(* Logix 5000 AddOnInstructionDefinition export GracoCore_DecodeDateTime; software revision 32.04; part 3 of 4 *)

ADD_ON_INSTRUCTION GracoPd2kDual_ReadFlushSeq   (* revision 1.0 *)
// Help:
// Returns the current configuration values for a flush sequence number.
// Values outside of acceptable ranges will result in an error being raised.
// State Codes:
// * 0000 (IDLE) - Idle
// * 1000 (BUSY) - Busy
// * 2000 (DONE) - Done
// * 4000 (ABORT) - Command overwritten by another process
// * 8000 (ERROR) - Flush sequence number out of range
// * 8001 (ERROR) - Timeout waiting for DCS registers
// * 8002 (ERROR) - Command unsuccessful
// * 8003 (ERROR) - Unhandled internal error
VAR_INPUT
   i_execute : BOOL; {visible}   // Execute command
   i_flushSeqNum : DINT; {visible}   // Flush sequence number
END_VAR
VAR_OUTPUT
   o_gunPurgeTime : DINT; {access Read Only, visible}   // Gun purge time (s)
   o_initialFlushVol : DINT; {access Read Only, visible}   // Initial flush volume (cc)
   o_finalFlushVol : DINT; {access Read Only, visible}   // Final flush volume (cc)
   o_numWashCycles : DINT; {access Read Only, visible}   // Number of wash cycles
   o_strokesPerWashCycle : DINT; {access Read Only, visible}   // Strokes per wash cycle
   o_busy : BOOL; {access Read Only, visible}   // Busy flag
   o_done : BOOL; {access Read Only, visible}   // Done flag
   o_aborted : BOOL; {access Read Only, visible}   // Aborted flag
   o_error : BOOL; {access Read Only, visible}   // Error flag
END_VAR
VAR_IN_OUT
   io_moduleStatus : DINT[62]; {required}   // Data from device to PLC
   io_moduleCmds : DINT[30]; {required}   // Data from PLC to device
END_VAR
VAR_OUTPUT
   o_state : DINT; {access Read Only, visible}   // Command state
END_VAR
VAR
   sendDCSInst : GracoPd2kDual_SendDCS; {access None}   // SendDCS instruction
END_VAR

ROUTINE Logic   (* ladder *)
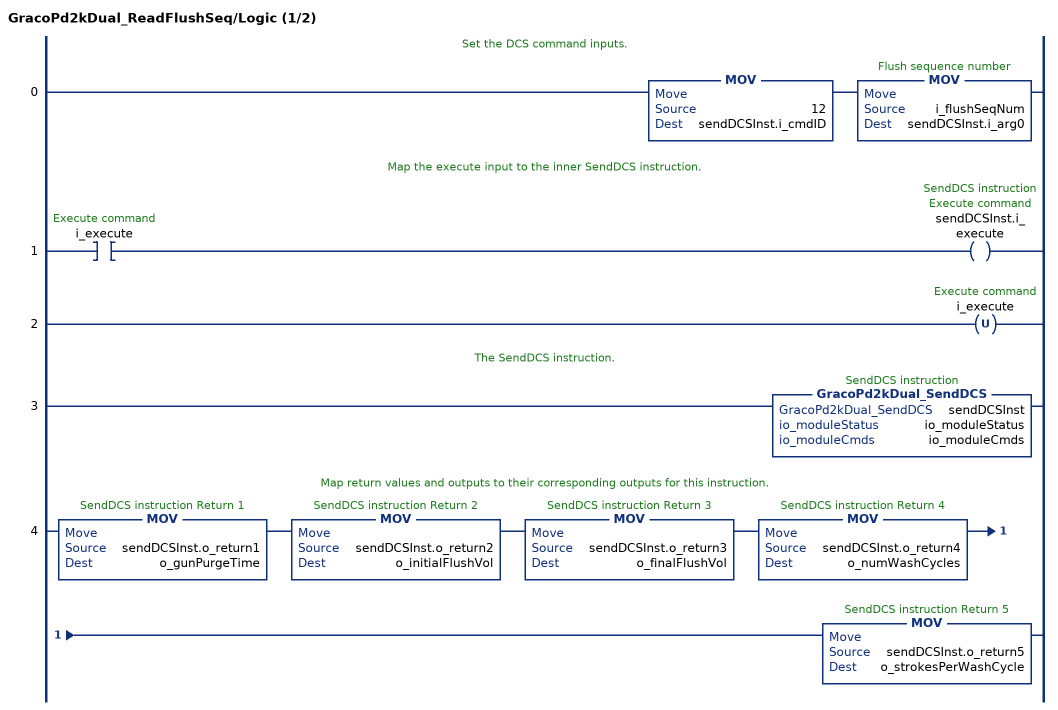
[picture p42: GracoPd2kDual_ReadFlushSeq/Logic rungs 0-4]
   // Set the DCS command inputs.
   0: MOV(12,sendDCSInst.i_cmdID)MOV(i_flushSeqNum,sendDCSInst.i_arg0);
   // Map the execute input to the inner SendDCS instruction.
   1: XIC(i_execute)OTE(sendDCSInst.i_execute);
   2: OTU(i_execute);
   // The SendDCS instruction.
   3: GracoPd2kDual_SendDCS(sendDCSInst,io_moduleStatus,io_moduleCmds);
   // Map return values and outputs to their corresponding outputs for this instruction.
   4: MOV(sendDCSInst.o_return1,o_gunPurgeTime)MOV(sendDCSInst.o_return2,o_initialFlushVol)MOV(sendDCSInst.o_return3,o_finalFlushVol)MOV(sendDCSInst.o_return4,o_numWashCycles)MOV(sendDCSInst.o_return5,o_strokesPerWashCycle);
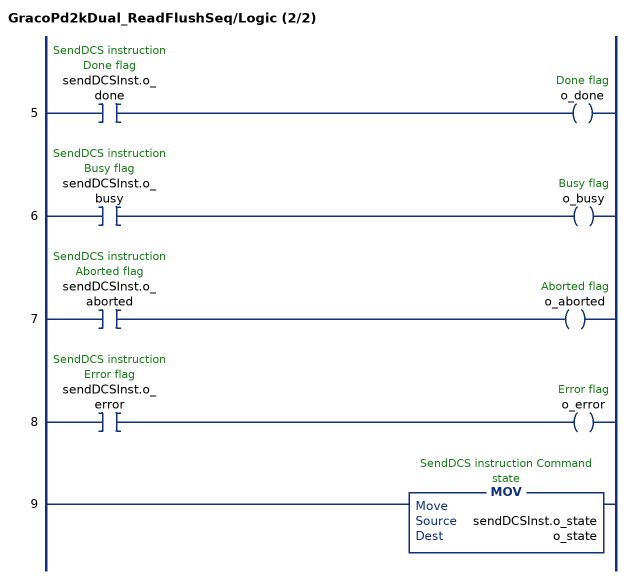
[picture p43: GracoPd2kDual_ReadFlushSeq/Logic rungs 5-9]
   5: XIC(sendDCSInst.o_done)OTE(o_done);
   6: XIC(sendDCSInst.o_busy)OTE(o_busy);
   7: XIC(sendDCSInst.o_aborted)OTE(o_aborted);
   8: XIC(sendDCSInst.o_error)OTE(o_error);
   9: MOV(sendDCSInst.o_state,o_state);
END_ROUTINE
END_ADD_ON_INSTRUCTION

ADD_ON_INSTRUCTION GracoPd2kDual_ReadGrandTotals   (* revision 1.0 *)
// Help:
// Returns the material usage statistics of the system.
// State Codes:
// * 0000 (IDLE) - Idle
// * 1000 (BUSY) - Busy
// * 2000 (DONE) - Done
// * 4000 (ABORT) - Command overwritten by another process
// * 8001 (ERROR) - Timeout waiting for DCS registers
// * 8002 (ERROR) - Command unsuccessful
// * 8003 (ERROR) - Unhandled internal error
VAR_INPUT
   i_execute : BOOL; {visible}   // Execute command
END_VAR
VAR_OUTPUT
   o_materialA : DINT; {access Read Only, visible}   // Material A total volume (gal)
   o_materialB : DINT; {access Read Only, visible}   // Material B total volume (gal)
   o_materialAB : DINT; {access Read Only, visible}   // Materials A+B total volume (gal)
   o_solvent : DINT; {access Read Only, visible}   // Solvent volume (gal)
   o_busy : BOOL; {access Read Only, visible}   // Busy flag
   o_done : BOOL; {access Read Only, visible}   // Done flag
   o_aborted : BOOL; {access Read Only, visible}   // Aborted flag
   o_error : BOOL; {access Read Only, visible}   // Error flag
   o_state : DINT; {access Read Only, visible}   // Command state
END_VAR
VAR_IN_OUT
   io_moduleStatus : DINT[62]; {required}   // Data from device to PLC
   io_moduleCmds : DINT[30]; {required}   // Data from PLC to device
END_VAR
VAR
   sendDCSInst : GracoPd2kDual_SendDCS; {access None}   // SendDCS instruction
END_VAR

ROUTINE Logic   (* ladder *)
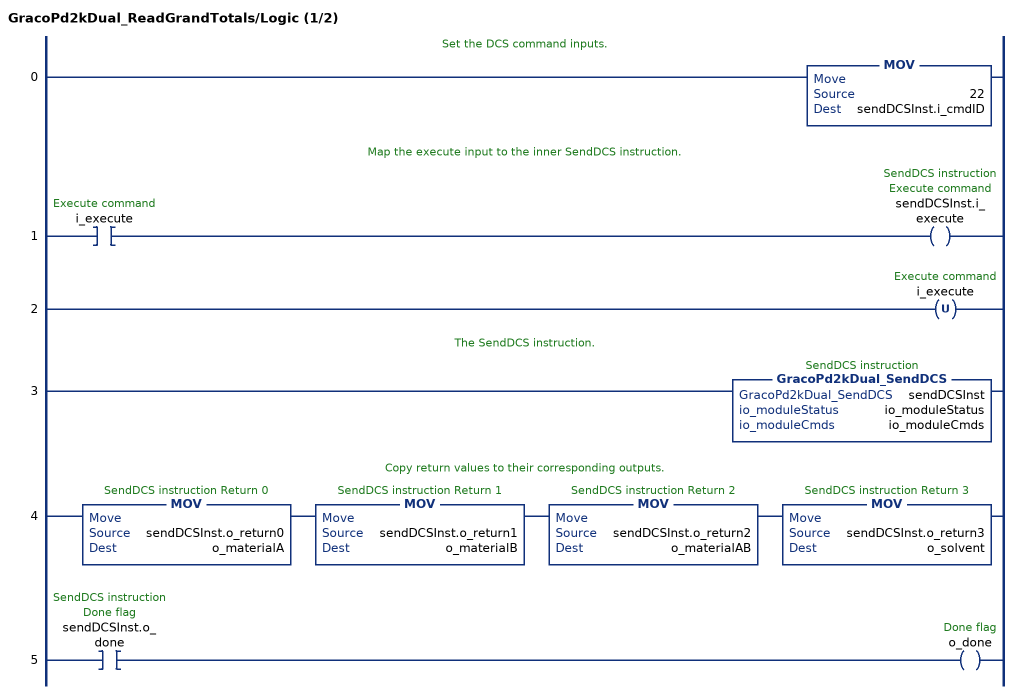
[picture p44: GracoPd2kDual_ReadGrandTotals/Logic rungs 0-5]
   // Set the DCS command inputs.
   0: MOV(22,sendDCSInst.i_cmdID);
   // Map the execute input to the inner SendDCS instruction.
   1: XIC(i_execute)OTE(sendDCSInst.i_execute);
   2: OTU(i_execute);
   // The SendDCS instruction.
   3: GracoPd2kDual_SendDCS(sendDCSInst,io_moduleStatus,io_moduleCmds);
   // Copy return values to their corresponding outputs.
   4: MOV(sendDCSInst.o_return0,o_materialA)MOV(sendDCSInst.o_return1,o_materialB)MOV(sendDCSInst.o_return2,o_materialAB)MOV(sendDCSInst.o_return3,o_solvent);
   5: XIC(sendDCSInst.o_done)OTE(o_done);
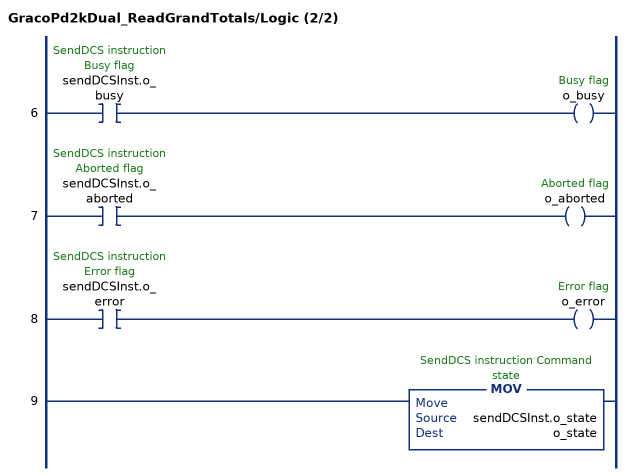
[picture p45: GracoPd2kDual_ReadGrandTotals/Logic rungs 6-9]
   6: XIC(sendDCSInst.o_busy)OTE(o_busy);
   7: XIC(sendDCSInst.o_aborted)OTE(o_aborted);
   8: XIC(sendDCSInst.o_error)OTE(o_error);
   9: MOV(sendDCSInst.o_state,o_state);
END_ROUTINE
END_ADD_ON_INSTRUCTION

ADD_ON_INSTRUCTION GracoPd2kDual_ReadRecipe   (* revision 1.0 *)
// Help:
// Returns the current configuration values for a recipe number.
// If mixUnitNum or recipeNum is out of range, an error will be raised.
// State Codes:
// * 0000 (IDLE) - Idle
// * 1000 (BUSY) - Busy
// * 2000 (DONE) - Done
// * 4000 (ABORT) - Command overwritten by another process
// * 8000 (ERROR) - Invalid input ranges
// * 8001 (ERROR) - Timeout waiting for DCS registers
// * 8002 (ERROR) - Command unsuccessful
// * 8003 (ERROR) - Unhandled internal error
VAR_INPUT
   i_execute : BOOL; {visible}   // Execute command
   i_mixUnitNum : DINT; {visible}   // Mix unit number (1-2)
   i_recipeNum : DINT; {visible}   // Recipe number (0-30)
END_VAR
VAR_OUTPUT
   o_materialA : DINT; {access Read Only, visible}   // Material A
   o_materialB : DINT; {access Read Only, visible}   // Material B
   o_flushSeqA : DINT; {access Read Only, visible}   // Flush sequence A
   o_flushSeqB : DINT; {access Read Only, visible}   // Flush sequence B
   o_mixRatioSP : REAL; {access Read Only, visible}   // Mix ratio setpoint (A:B)
   o_potLifeTimeSP : DINT; {access Read Only, visible}   // Pot life time setpoint (min)
   o_mixPressureTol : DINT; {access Read Only, visible}   // Mix pressure tolerance (%)
   o_busy : BOOL; {access Read Only, visible}   // Busy flag
   o_done : BOOL; {access Read Only, visible}   // Done flag
   o_aborted : BOOL; {access Read Only, visible}   // Aborted flag
   o_error : BOOL; {access Read Only, visible}   // Error flag
   o_state : DINT; {access Read Only, visible}   // Command state
END_VAR
VAR_IN_OUT
   io_moduleStatus : DINT[62]; {required}   // Data from device to PLC
   io_moduleCmds : DINT[30]; {required}   // Data from PLC to device
END_VAR
VAR
   sendDCSInst : GracoPd2kDual_SendDCS; {access None}   // SendDCS instruction
END_VAR

ROUTINE Logic   (* ladder *)
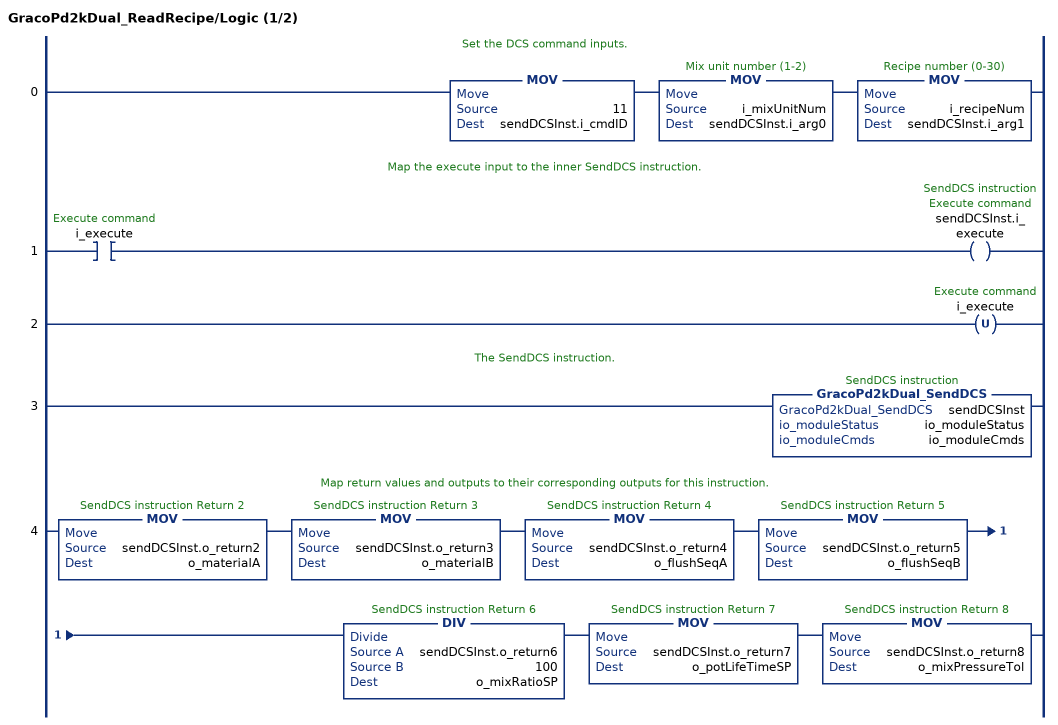
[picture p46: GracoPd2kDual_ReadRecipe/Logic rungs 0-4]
   // Set the DCS command inputs.
   0: MOV(11,sendDCSInst.i_cmdID)MOV(i_mixUnitNum,sendDCSInst.i_arg0)MOV(i_recipeNum,sendDCSInst.i_arg1);
   // Map the execute input to the inner SendDCS instruction.
   1: XIC(i_execute)OTE(sendDCSInst.i_execute);
   2: OTU(i_execute);
   // The SendDCS instruction.
   3: GracoPd2kDual_SendDCS(sendDCSInst,io_moduleStatus,io_moduleCmds);
   // Map return values and outputs to their corresponding outputs for this instruction.
   4: MOV(sendDCSInst.o_return2,o_materialA)MOV(sendDCSInst.o_return3,o_materialB)MOV(sendDCSInst.o_return4,o_flushSeqA)MOV(sendDCSInst.o_return5,o_flushSeqB)DIV(sendDCSInst.o_return6,100,o_mixRatioSP)MOV(sendDCSInst.o_return7,o_potLifeTimeSP)MOV(sendDCSInst.o_return8,o_mixPressureTol);
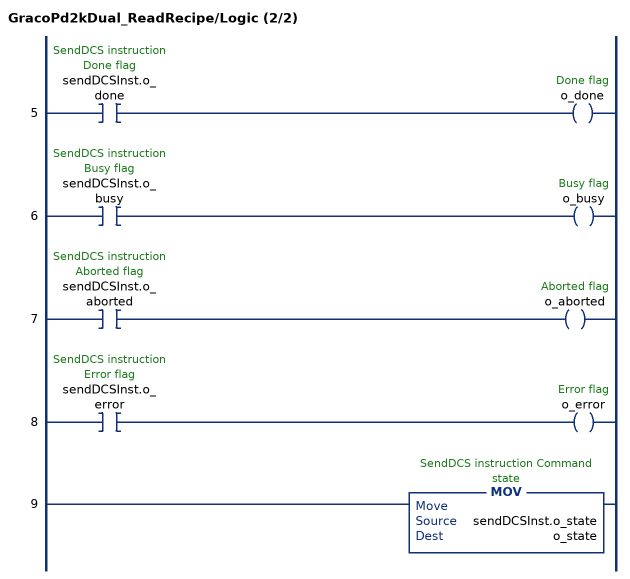
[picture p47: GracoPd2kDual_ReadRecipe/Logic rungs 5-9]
   5: XIC(sendDCSInst.o_done)OTE(o_done);
   6: XIC(sendDCSInst.o_busy)OTE(o_busy);
   7: XIC(sendDCSInst.o_aborted)OTE(o_aborted);
   8: XIC(sendDCSInst.o_error)OTE(o_error);
   9: MOV(sendDCSInst.o_state,o_state);
END_ROUTINE
END_ADD_ON_INSTRUCTION

ADD_ON_INSTRUCTION GracoPd2kDual_RecipeChange   (* revision 1.0 *)
// Help:
// Performs a recipe change operation.
// This command monitors the system throughout the operation, returning state codes depending on various conditions.
// State Codes:
// * 0000 (IDLE) - Idle
// * 1000 (BUSY) - busy
// * 2000 (DONE) - Complete
// * 4000 (ABORT) - Command overwritten by another process
// * 8000 (ERROR) - Invalid input ranges
// * 8001 (ERROR) - Could not start, pumps are turned off
// * 8002 (ERROR) - Another recipe change is currently in progress
// * 8003 (ERROR) - Could not start, a system alarm in active
// * 8004 (ERROR) - Could not start, another operation is in progress
// * 8006 (ERROR) - Timeout waiting for DCS registers
// * 8007 (ERROR) - Alarm occurred
// * 8008 (ERROR) - Unexpected system mode
// * 8009 (ERROR) - Timeout occurred waiting for fill to start
// * 800A (ERROR) - Timeout occurred waiting for mixing to start
// * 800B (ERROR) - Timeout occurred waiting for system command register
VAR_INPUT
   i_execute : BOOL; {visible}   // Execute command
   i_recipeNum : DINT; {visible}   // Recipe number
   i_mixUnitNum : DINT; {visible}   // Mix unit number
END_VAR
VAR_IN_OUT
   io_moduleStatus : DINT[62]; {required}   // Data from device to PLC
   io_moduleCmds : DINT[30]; {required}   // Data from PLC to device
END_VAR
VAR_OUTPUT
   o_busy : BOOL; {access Read Only, visible}   // Busy flag
   o_done : BOOL; {access Read Only, visible}   // Done flag
   o_aborted : BOOL; {access Read Only, visible}   // Aborted flag
   o_error : BOOL; {access Read Only, visible}   // Error flag
   o_state : DINT; {access Read Only, visible}   // Command state
END_VAR
VAR
   _systemMode : DINT; {access None}   // Current system mode
   rateLimitTmr : TIMER := (PRE := 250); {access None}   // Rate limit timer
   state_writeGotoRecipe : DINT; {access None}
   state_writeCmd : DINT; {access None}
   state_rateLimit : DINT; {access None}
   state_errorUnknownSystemMode : DINT; {access None}
   state_errorSystemInUse : DINT; {access None}
   state_errorRecipeChangeInProgress : DINT; {access None}
   state_errorPowerIsOff : DINT; {access None}
   state_errorIncomplete : DINT; {access None}
   state_errorAnotherOperation : DINT; {access None}
   state_errorAlarmOccurred : DINT; {access None}
   state_errorAlarmActive : DINT; {access None}
   state_done : DINT; {access None}
   state_checkSysState : DINT; {access None}
   state_await : DINT; {access None}
   state_aborted : DINT; {access None}
   recipeCmdConstant : DINT; {access None}
   _nextState : DINT; {access None}
   recipeChangeInProgress : BOOL; {access None}
   inStandby : BOOL; {access None}
   knownSystemMode : BOOL; {access None}
   systemPowerIsOff : BOOL; {access None}
   alarmIsActive : BOOL; {access None}
   systemInMixReadyMode : BOOL; {access None}
   systemInFillReadyMode : BOOL; {access None}
   systemInMixNotReadyMode : BOOL; {access None}
   state_checkInputs : DINT; {access None}
   _mixUnitNum : DINT; {access None}   // Mix unit number (internal)
   inUseTmr : TIMER := (PRE := 5000); {access None}
   recipeNumDelayTmr : TIMER := (PRE := 200); {access None}
   startedTmr : TIMER := (PRE := 2000); {access None}
   recipeChangeCompleted : BOOL; {access None}
   incompleteStuckInFillReady : BOOL; {access None}
   incompleteMixNotReady : BOOL; {access None}
   incompleteUnexpectedMode : BOOL; {access None}
   execute_ons : BOOL; {access None}
   mixUnitNumIsValid : BOOL; {access None}
   state_errorInvalidMixUnitNum : DINT; {access None}
   _currentSystemCmd : DINT; {access None}
   _currentNextRecipeCmd : DINT; {access None}
END_VAR

ROUTINE Logic   (* ladder *)
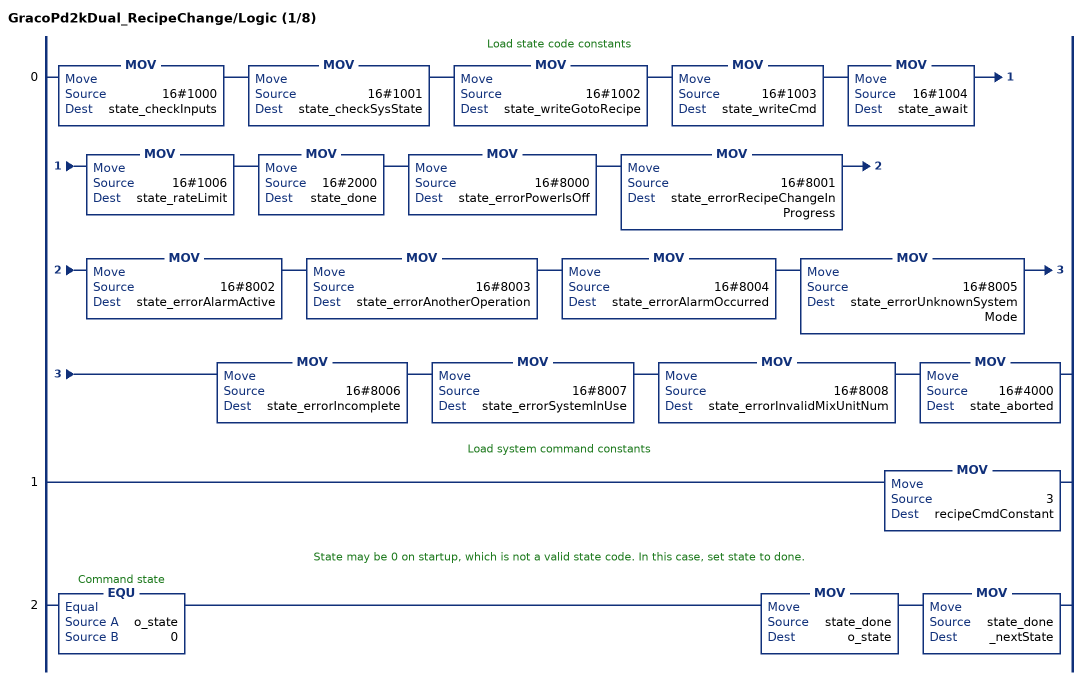
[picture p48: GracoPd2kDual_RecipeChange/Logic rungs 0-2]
   // Load state code constants
   0: MOV(16#1000,state_checkInputs)MOV(16#1001,state_checkSysState)MOV(16#1002,state_writeGotoRecipe)MOV(16#1003,state_writeCmd)MOV(16#1004,state_await)MOV(16#1006,state_rateLimit)MOV(16#2000,state_done)MOV(16#8000,state_errorPowerIsOff)MOV(16#8001,state_errorRecipeChangeInProgress)MOV(16#8002,state_errorAlarmActive)MOV(16#8003,state_errorAnotherOperation)MOV(16#8004,state_errorAlarmOccurred)MOV(16#8005,state_errorUnknownSystemMode)MOV(16#8006,state_errorIncomplete)MOV(16#8007,state_errorSystemInUse)MOV(16#8008,state_errorInvalidMixUnitNum)MOV(16#4000,state_aborted);
   // Load system command constants
   1: MOV(3,recipeCmdConstant);
   // State may be 0 on startup, which is not a valid state code. In this case, set state to done.
   2: EQU(o_state,0)MOV(state_done,o_state)MOV(state_done,_nextState);
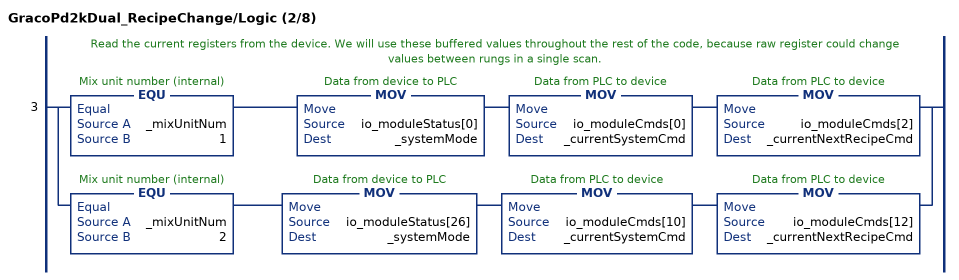
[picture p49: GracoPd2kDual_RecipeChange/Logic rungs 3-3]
   // Read the current registers from the device. We will use these buffered values throughout the rest of the code, because raw register could change values between rungs in a single scan.
   3: [EQU(_mixUnitNum,1) MOV(io_moduleStatus[0],_systemMode) MOV(io_moduleCmds[0],_currentSystemCmd) MOV(io_moduleCmds[2],_currentNextRecipeCmd) ,EQU(_mixUnitNum,2) MOV(io_moduleStatus[26],_systemMode) MOV(io_moduleCmds[10],_currentSystemCmd) MOV(io_moduleCmds[12],_currentNextRecipeCmd) ];
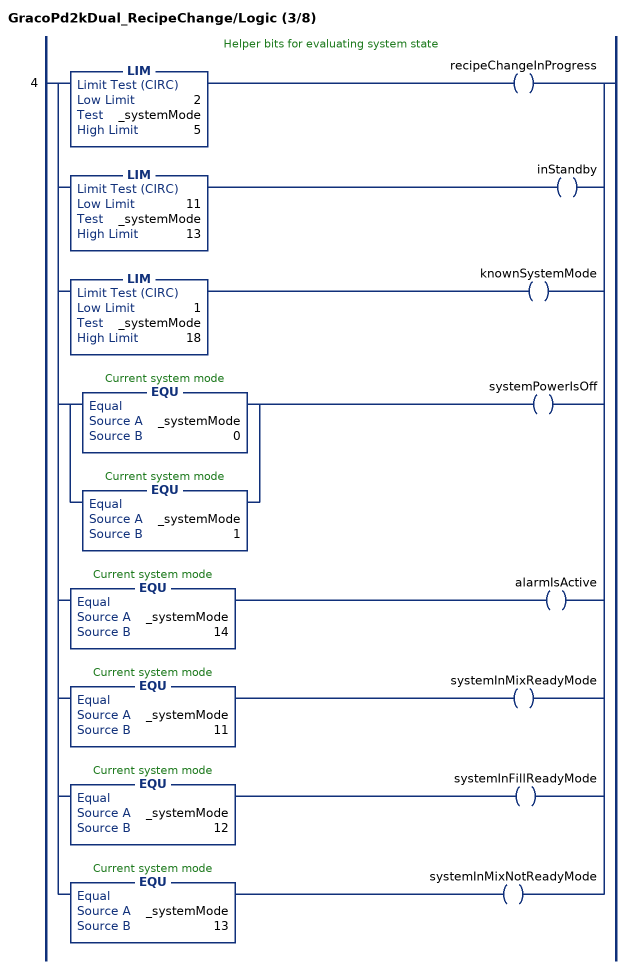
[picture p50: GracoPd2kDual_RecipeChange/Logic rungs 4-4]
   // Helper bits for evaluating system state
   4: [LIM(2,_systemMode,5) OTE(recipeChangeInProgress) ,LIM(11,_systemMode,13) OTE(inStandby) ,LIM(1,_systemMode,18) OTE(knownSystemMode) ,[EQU(_systemMode,0) ,EQU(_systemMode,1) ] OTE(systemPowerIsOff) ,EQU(_systemMode,14) OTE(alarmIsActive) ,EQU(_systemMode,11) OTE(systemInMixReadyMode) ,EQU(_systemMode,12) OTE(systemInFillReadyMode) ,EQU(_systemMode,13) OTE(systemInMixNotReadyMode) ];
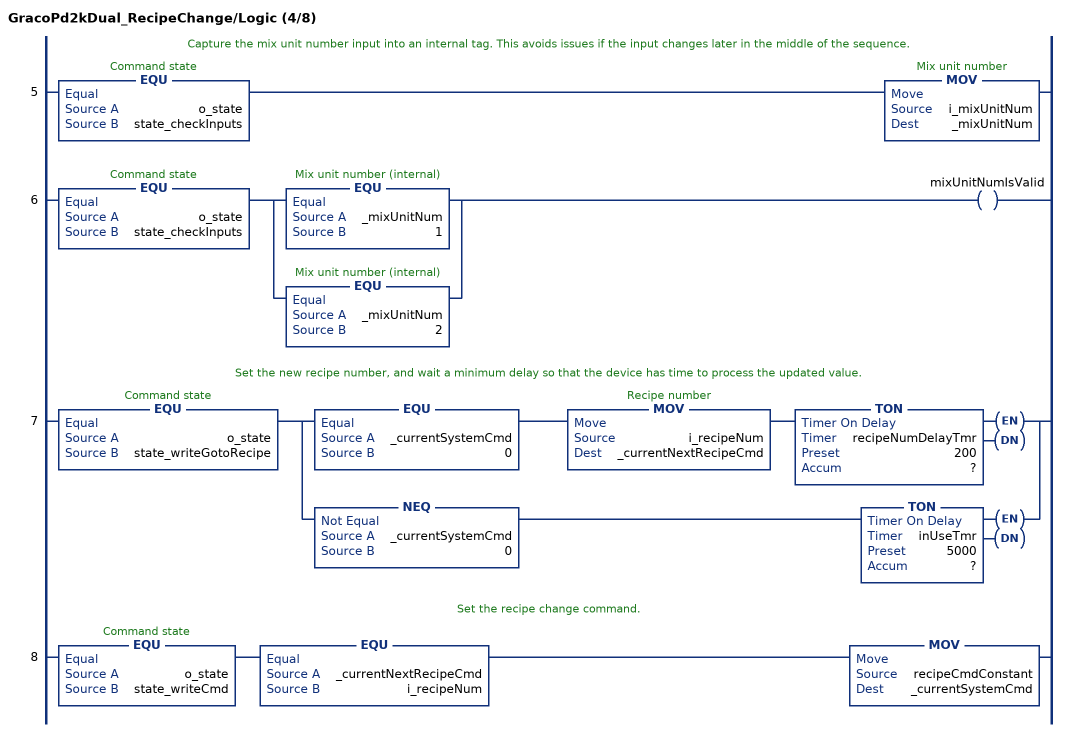
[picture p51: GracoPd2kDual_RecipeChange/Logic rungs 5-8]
   // Capture the mix unit number input into an internal tag. This avoids issues if the input changes later in the middle of the sequence.
   5: EQU(o_state,state_checkInputs)MOV(i_mixUnitNum,_mixUnitNum);
   6: EQU(o_state,state_checkInputs)[EQU(_mixUnitNum,1) ,EQU(_mixUnitNum,2) ]OTE(mixUnitNumIsValid);
   // Set the new recipe number, and wait a minimum delay so that the device has time to process the updated value.
   7: EQU(o_state,state_writeGotoRecipe)[EQU(_currentSystemCmd,0) MOV(i_recipeNum,_currentNextRecipeCmd) TON(recipeNumDelayTmr,?,?) ,NEQ(_currentSystemCmd,0) TON(inUseTmr,?,?) ];
   // Set the recipe change command.
   8: EQU(o_state,state_writeCmd)EQU(_currentNextRecipeCmd,i_recipeNum)MOV(recipeCmdConstant,_currentSystemCmd);
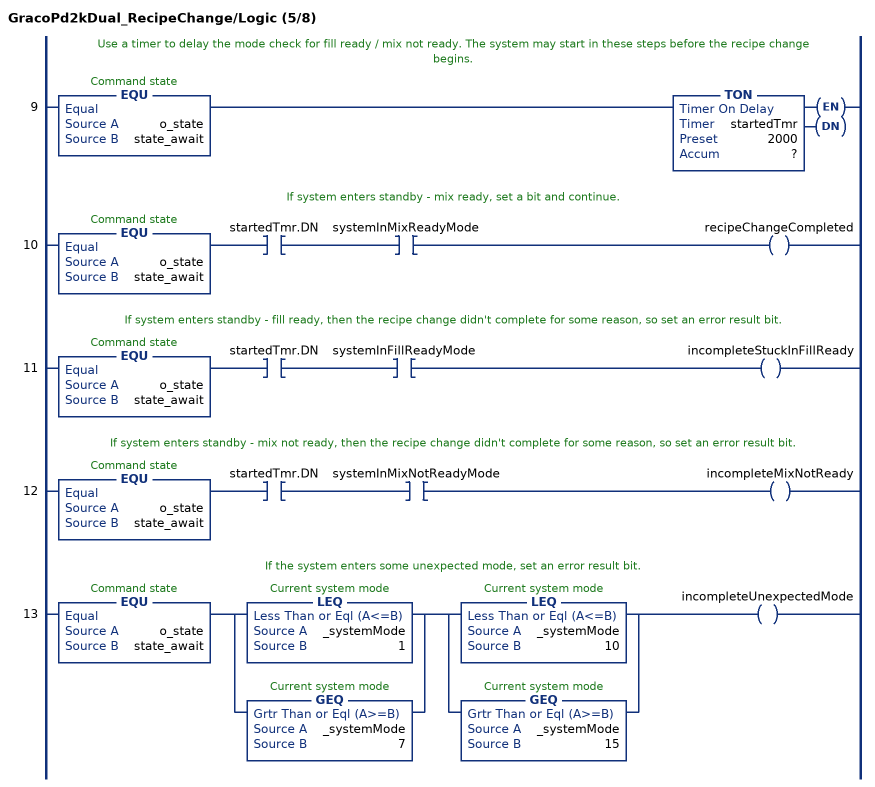
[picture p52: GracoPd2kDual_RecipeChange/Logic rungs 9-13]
   // Use a timer to delay the mode check for fill ready / mix not ready. The system may start in these steps before the recipe change begins.
   9: EQU(o_state,state_await)TON(startedTmr,?,?);
   // If system enters standby - mix ready, set a bit and continue.
   10: EQU(o_state,state_await)XIC(startedTmr.DN)XIC(systemInMixReadyMode)OTE(recipeChangeCompleted);
   // If system enters standby - fill ready, then the recipe change didn't complete for some reason, so set an error result bit.
   11: EQU(o_state,state_await)XIC(startedTmr.DN)XIC(systemInFillReadyMode)OTE(incompleteStuckInFillReady);
   // If system enters standby - mix not ready, then the recipe change didn't complete for some reason, so set an error result bit.
   12: EQU(o_state,state_await)XIC(startedTmr.DN)XIC(systemInMixNotReadyMode)OTE(incompleteMixNotReady);
   // If the system enters some unexpected mode, set an error result bit.
   13: EQU(o_state,state_await)[LEQ(_systemMode,1) ,GEQ(_systemMode,7) ][LEQ(_systemMode,10) ,GEQ(_systemMode,15) ]OTE(incompleteUnexpectedMode);
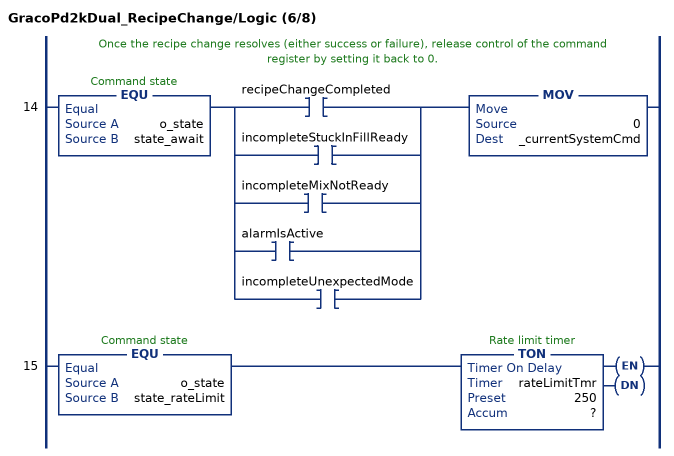
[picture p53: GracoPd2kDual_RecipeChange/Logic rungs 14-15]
   // Once the recipe change resolves (either success or failure), release control of the command register by setting it back to 0.
   14: EQU(o_state,state_await)[XIC(recipeChangeCompleted) ,XIC(incompleteStuckInFillReady) ,XIC(incompleteMixNotReady) ,XIC(alarmIsActive) ,XIC(incompleteUnexpectedMode) ]MOV(0,_currentSystemCmd);
   15: EQU(o_state,state_rateLimit)TON(rateLimitTmr,?,?);
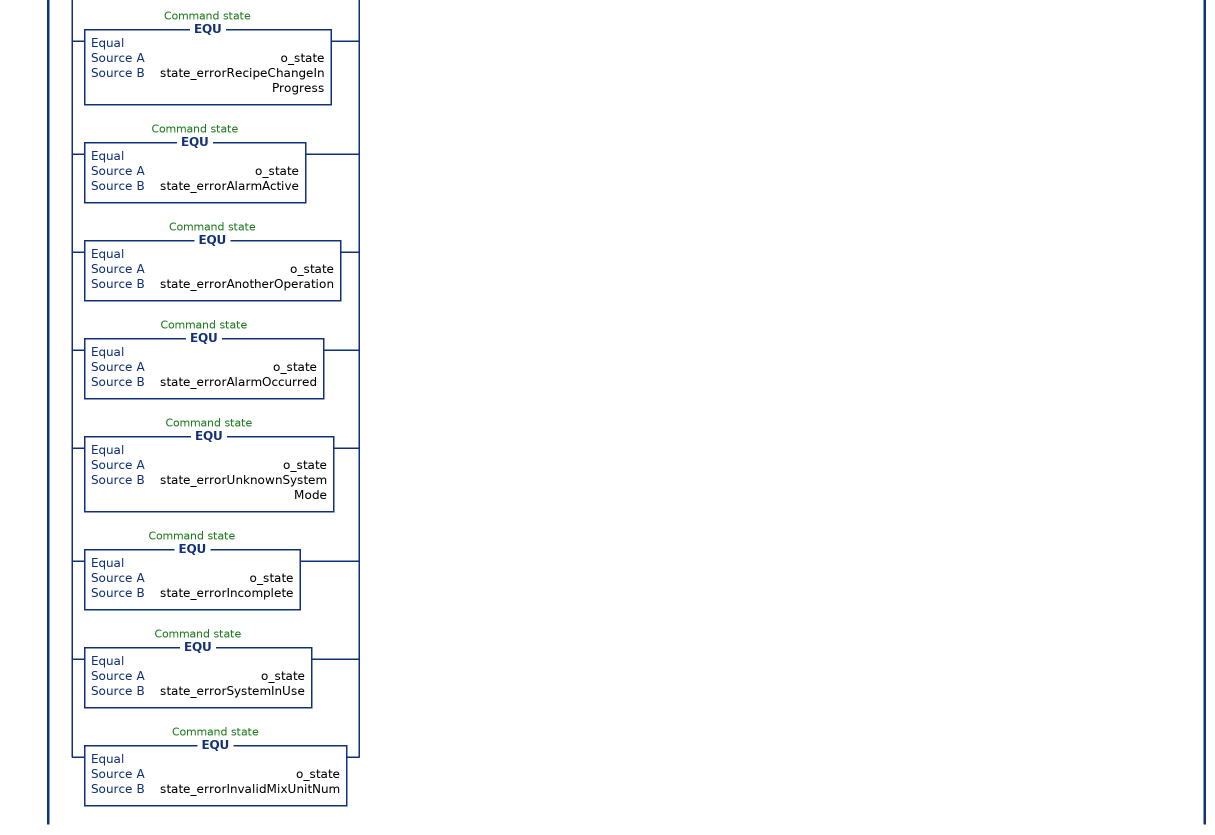
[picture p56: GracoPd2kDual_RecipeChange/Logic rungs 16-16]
   // Advance the state machine
   16: [EQU(o_state,state_checkInputs) [XIC(mixUnitNumIsValid) MOV(state_checkSysState,_nextState) ,XIO(mixUnitNumIsValid) MOV(state_errorInvalidMixUnitNum,_nextState) ] ,EQU(o_state,state_checkSysState) [XIC(systemPowerIsOff) MOV(state_errorPowerIsOff,_nextState) ,XIC(recipeChangeInProgress) MOV(state_errorRecipeChangeInProgress,_nextState) ,XIC(inStandby) MOV(state_writeGotoRecipe,_nextState) ,XIC(alarmIsActive) MOV(state_errorAlarmActive,_nextState) ,XIC(knownSystemMode) XIO(systemPowerIsOff) XIO(alarmIsActive) XIO(recipeChangeInProgress) XIO(inStandby) MOV(state_errorAnotherOperation,_nextState) ,XIO(knownSystemMode) MOV(state_errorUnknownSystemMode,_nextState) ] ,EQU(o_state,state_writeGotoRecipe) [XIC(recipeNumDelayTmr.DN) MOV(state_writeCmd,_nextState) ,XIC(inUseTmr.DN) MOV(state_errorSystemInUse,_nextState) ] ,EQU(o_state,state_writeCmd) [EQU(_currentSystemCmd,recipeCmdConstant) MOV(state_await,_nextState) ,NEQ(_currentNextRecipeCmd,i_recipeNum) MOV(state_writeGotoRecipe,_nextState) ] ,EQU(o_state,state_await) [NEQ(_currentSystemCmd,recipeCmdConstant) MOV(state_aborted,_nextState) ,XIC(recipeChangeCompleted) MOV(state_rateLimit,_nextState) ,[XIC(incompleteMixNotReady) ,XIC(incompleteStuckInFillReady) ,XIC(incompleteUnexpectedMode) ] MOV(state_errorIncomplete,_nextState) ,XIC(alarmIsActive) MOV(state_errorAlarmOccurred,_nextState) ] ,EQU(o_state,state_rateLimit) XIC(rateLimitTmr.DN) MOV(state_done,_nextState) ,[EQU(o_state,state_done) ,EQU(o_state,state_aborted) ,EQU(o_state,state_errorPowerIsOff) ,EQU(o_state,state_errorRecipeChangeInProgress) ,EQU(o_state,state_errorAlarmActive) ,EQU(o_state,state_errorAnotherOperation) ,EQU(o_state,state_errorAlarmOccurred) ,EQU(o_state,state_errorUnknownSystemMode) ,EQU(o_state,state_errorIncomplete) ,EQU(o_state,state_errorSystemInUse) ,EQU(o_state,state_errorInvalidMixUnitNum) ] XIC(i_execute) ONS(execute_ons) MOV(state_checkInputs,_nextState) ];
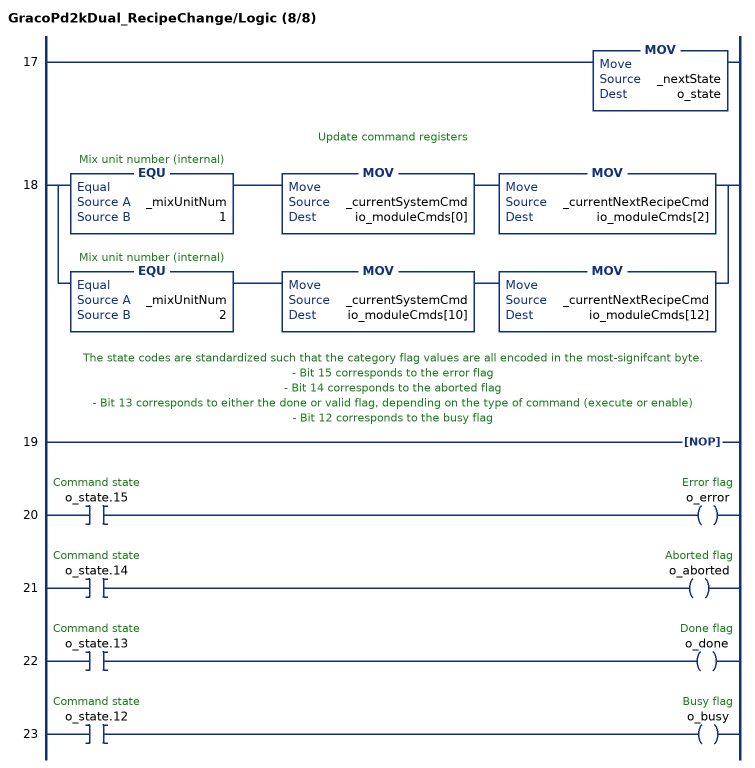
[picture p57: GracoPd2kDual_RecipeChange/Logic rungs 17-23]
   17: MOV(_nextState,o_state);
   // Update command registers
   18: [EQU(_mixUnitNum,1) MOV(_currentSystemCmd,io_moduleCmds[0]) MOV(_currentNextRecipeCmd,io_moduleCmds[2]) ,EQU(_mixUnitNum,2) MOV(_currentSystemCmd,io_moduleCmds[10]) MOV(_currentNextRecipeCmd,io_moduleCmds[12]) ];
   // The state codes are standardized such that the category flag values are all encoded in the most-signifcant byte.
   // - Bit 15 corresponds to the error flag
   // - Bit 14 corresponds to the aborted flag
   // - Bit 13 corresponds to either the done or valid flag, depending on the type of command (execute or enable)
   // - Bit 12 corresponds to the busy flag
   19: NOP();
   20: XIC(o_state.15)OTE(o_error);
   21: XIC(o_state.14)OTE(o_aborted);
   22: XIC(o_state.13)OTE(o_done);
   23: XIC(o_state.12)OTE(o_busy);
END_ROUTINE
END_ADD_ON_INSTRUCTION

ADD_ON_INSTRUCTION GracoPd2kDual_WriteFlushSeq   (* revision 1.0 *)
// Help:
// Configures the values for a flush sequence number.
// Values outside of acceptable ranges will result in an error being raised.
// State Codes:
// * 0000 (IDLE) - Idle
// * 1000 (BUSY) - Busy
// * 2000 (DONE) - Done
// * 4000 (ABORT) - Command overwritten by another process
// * 8000 (ERROR) - Flush sequence number out of range
// * 8001 (ERROR) - Timeout waiting for DCS registers
// * 8002 (ERROR) - Command unsuccessful
// * 8003 (ERROR) - Unhandled internal error
VAR_INPUT
   i_execute : BOOL; {visible}   // Execute command
   i_flushSeqNum : DINT; {visible}   // Flush sequence number
   i_gunPurgeTime : DINT; {visible}   // Gun purge time (s)
   i_initialFlushVol : DINT; {visible}   // Initial flush volume (cc)
   i_finalFlushVol : DINT; {visible}   // Final flush volume (cc)
   i_numWashCycles : DINT; {visible}   // Number of wash cycles
   i_strokesPerWashCycle : DINT; {visible}   // Strokes per wash cycle
END_VAR
VAR_OUTPUT
   o_busy : BOOL; {access Read Only, visible}   // Busy flag
   o_done : BOOL; {access Read Only, visible}   // Done flag
   o_aborted : BOOL; {access Read Only, visible}   // Aborted flag
   o_error : BOOL; {access Read Only, visible}   // Error flag
   o_state : DINT; {access Read Only, visible}   // Command state
END_VAR
VAR_IN_OUT
   io_moduleStatus : DINT[62]; {required}   // Data from device to PLC
   io_moduleCmds : DINT[30]; {required}   // Data from PLC to device
END_VAR
VAR
   sendDCSInst : GracoPd2kDual_SendDCS; {access None}   // SendDCS instruction
END_VAR

ROUTINE Logic   (* ladder *)
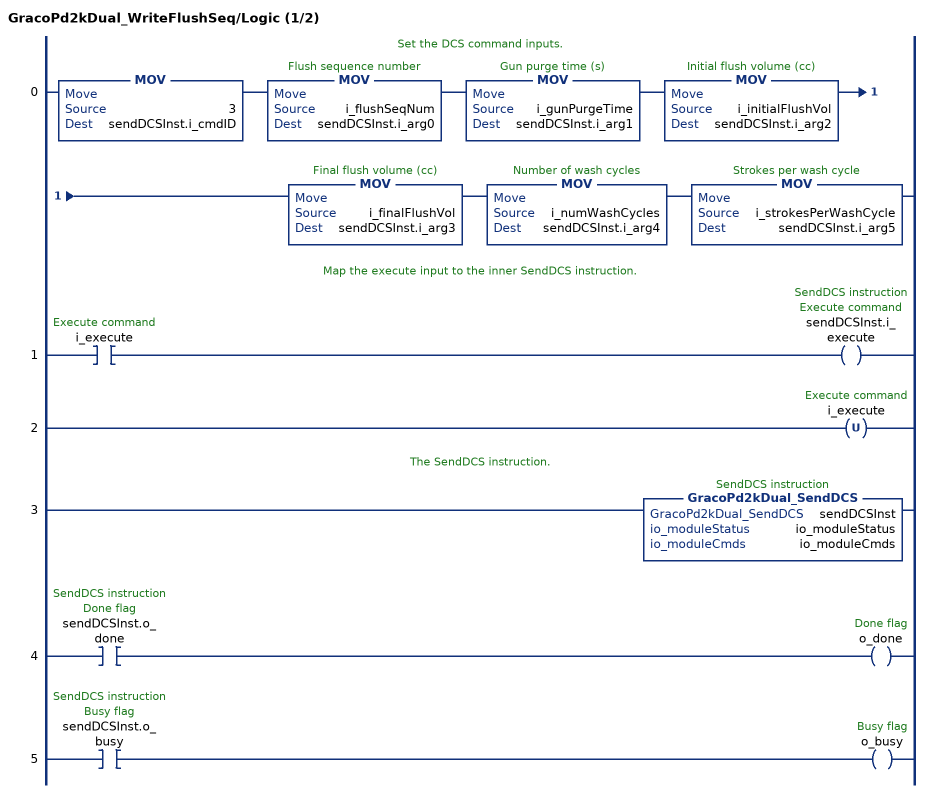
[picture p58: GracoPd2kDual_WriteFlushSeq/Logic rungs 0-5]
   // Set the DCS command inputs.
   0: MOV(3,sendDCSInst.i_cmdID)MOV(i_flushSeqNum,sendDCSInst.i_arg0)MOV(i_gunPurgeTime,sendDCSInst.i_arg1)MOV(i_initialFlushVol,sendDCSInst.i_arg2)MOV(i_finalFlushVol,sendDCSInst.i_arg3)MOV(i_numWashCycles,sendDCSInst.i_arg4)MOV(i_strokesPerWashCycle,sendDCSInst.i_arg5);
   // Map the execute input to the inner SendDCS instruction.
   1: XIC(i_execute)OTE(sendDCSInst.i_execute);
   2: OTU(i_execute);
   // The SendDCS instruction.
   3: GracoPd2kDual_SendDCS(sendDCSInst,io_moduleStatus,io_moduleCmds);
   4: XIC(sendDCSInst.o_done)OTE(o_done);
   5: XIC(sendDCSInst.o_busy)OTE(o_busy);
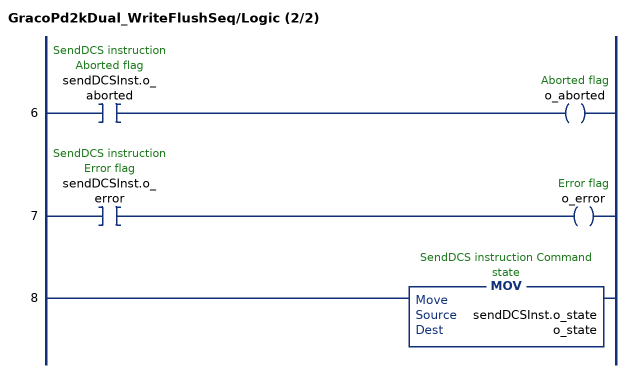
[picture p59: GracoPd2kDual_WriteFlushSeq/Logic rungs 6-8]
   6: XIC(sendDCSInst.o_aborted)OTE(o_aborted);
   7: XIC(sendDCSInst.o_error)OTE(o_error);
   8: MOV(sendDCSInst.o_state,o_state);
END_ROUTINE
END_ADD_ON_INSTRUCTION

ADD_ON_INSTRUCTION GracoPd2kDual_WriteMaterialReadyFlag   (* revision 1.0 *)
// Help:
// Sets the material ready flag, which is used to signal the state of upstream material management to the PD2K.
// This flag is only used when multiple material for a pump are fed to the PD2K via a single valve at the inlet valve stack (i.e. a piggable system). For more information, see the system operation manual.
// State Codes:
// * 0000 (IDLE) - Idle
// * 1000 (BUSY) - Busy
// * 2000 (DONE) - Done
// * 4000 (ABORT) - Command overwritten by another process
// * 8000 (ERROR) - Mix unit number out of range
// * 8001 (ERROR) - Timeout waiting for DCS registers
// * 8002 (ERROR) - Command unsuccessful
// * 8003 (ERROR) - Unhandled internal error
VAR_INPUT
   i_mixUnitNum : DINT; {visible}   // Mix unit number
   i_execute : BOOL; {visible}   // Execute command
   i_materialReadyFlag : BOOL; {visible}   // Material ready flag
END_VAR
VAR_OUTPUT
   o_busy : BOOL; {access Read Only, visible}   // Busy flag
   o_done : BOOL; {access Read Only, visible}   // Done flag
   o_aborted : BOOL; {access Read Only, visible}   // Aborted flag
   o_error : BOOL; {access Read Only, visible}   // Error flag
END_VAR
VAR_IN_OUT
   io_moduleStatus : DINT[62]; {required}   // Data from device to PLC
   io_moduleCmds : DINT[30]; {required}   // Data from PLC to device
END_VAR
VAR_OUTPUT
   o_state : DINT; {access Read Only, visible}   // Command state
END_VAR
VAR
   sendDCSInst : GracoPd2kDual_SendDCS; {access None}   // SendDCS instruction
END_VAR

ROUTINE Logic   (* ladder *)
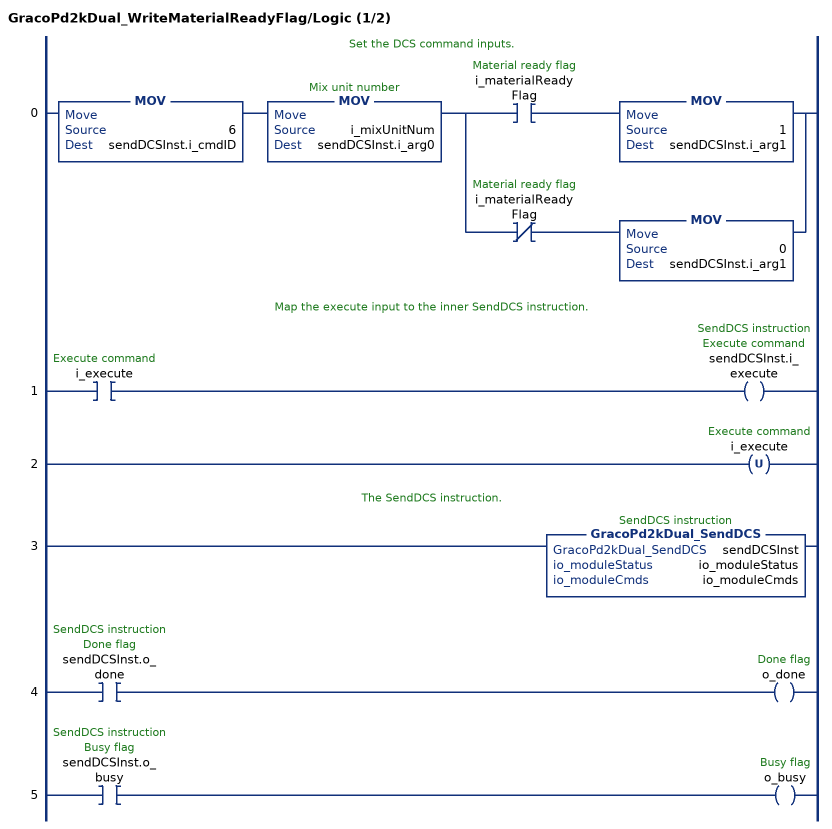
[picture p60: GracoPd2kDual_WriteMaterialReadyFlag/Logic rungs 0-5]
   // Set the DCS command inputs.
   0: MOV(6,sendDCSInst.i_cmdID)MOV(i_mixUnitNum,sendDCSInst.i_arg0)[XIC(i_materialReadyFlag) MOV(1,sendDCSInst.i_arg1) ,XIO(i_materialReadyFlag) MOV(0,sendDCSInst.i_arg1) ];
   // Map the execute input to the inner SendDCS instruction.
   1: XIC(i_execute)OTE(sendDCSInst.i_execute);
   2: OTU(i_execute);
   // The SendDCS instruction.
   3: GracoPd2kDual_SendDCS(sendDCSInst,io_moduleStatus,io_moduleCmds);
   4: XIC(sendDCSInst.o_done)OTE(o_done);
   5: XIC(sendDCSInst.o_busy)OTE(o_busy);
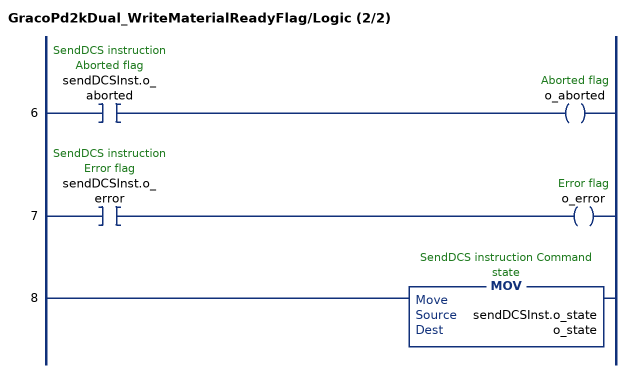
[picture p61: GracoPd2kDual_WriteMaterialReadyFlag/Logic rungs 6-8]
   6: XIC(sendDCSInst.o_aborted)OTE(o_aborted);
   7: XIC(sendDCSInst.o_error)OTE(o_error);
   8: MOV(sendDCSInst.o_state,o_state);
END_ROUTINE
END_ADD_ON_INSTRUCTION
